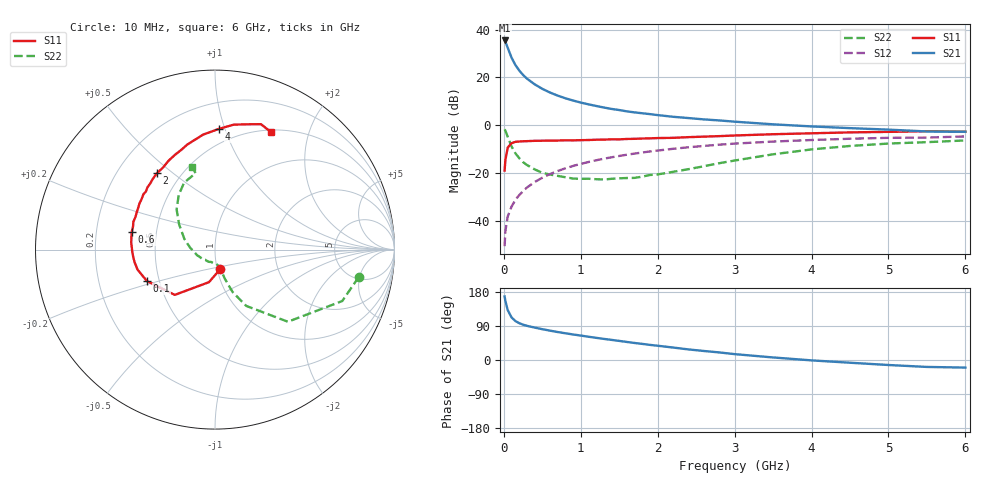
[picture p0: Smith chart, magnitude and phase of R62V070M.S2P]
! SIEMENS Small Signal Semiconductors
! BFR193
! Si NPN RF Bipolar Junction Transistor in SOT23
! VCE = 2 V  IC = 70 mA
! Common Emitter S-Parameters:  May  1996
# GHz  S  MA  R  50
!  f  S11  S21  S12  S22
! GHz  MAG  ANG  MAG  ANG  MAG  ANG  MAG  ANG
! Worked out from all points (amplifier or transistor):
!   36 points, 10 MHz to 6 GHz, reference 50 ohm
!   highest |S21| = 35.5 dB at 10 MHz (marker M1)
!   |S21| within 3 dB of that: start of sweep to 49.59 MHz
!   unconditionally stable (mu >= 1): 227.5 MHz to 2.247 GHz
!   at 250 MHz: K = 1.01, MAG = 23.6 dB, |S12| = -27.7 dB
!   at 1.4 GHz: K = 1.03, MAG = 9.0 dB, |S12| = -13.5 dB
!   at 6 GHz: K = 0.98, MSG = 1.0 dB, |S12| = -4.7 dB
!   S11 on the Smith chart (normalised r, x): 10 MHz: 1.04, -0.23; 100 MHz: 0.43, -0.18; 600 MHz: 0.36, +0.09; 2 GHz: 0.37, +0.44; 4 GHz: 0.39, +0.96; 6 GHz: 0.52, +1.45
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0.01  0.1114 -74.2  59.45 167.6  0.0029 79.5  0.8152 -10.8
0.02  0.1843 -100.4  56.14 156.1  0.006 72.3  0.7648 -22.0
0.05  0.3373 -131.6  41.92 131.8  0.0121 69.0  0.5715 -44.7
0.1  0.4179 -155.2  25.99 112.4  0.0195 69.5  0.3586 -61.0
0.15  0.4456 -165.5  18.21 102.8  0.0271 71.9  0.2568 -67.4
0.2  0.4536 -171.1  13.97 97.2  0.0341 74.3  0.2032 -69.6
0.25  0.4578 -175.2  11.25 93.2  0.0413 74.9  0.1675 -71.5
0.3  0.461 -178.6  9.426 90.2  0.0491 75.7  0.1462 -72.3
0.4  0.4683 175.3  7.171 85.6  0.0641 75.6  0.1181 -74.1
0.5  0.4705 172.1  5.76 81.3  0.0788 75.1  0.1001 -75.4
0.6  0.4743 167.9  4.817 77.5  0.094 73.9  0.0919 -77.7
0.7  0.4744 164.2  4.149 73.8  0.109 72.9  0.0863 -81.1
0.8  0.4804 161.3  3.65 70.5  0.1243 71.5  0.0806 -84.5
1.1  0.4868 151.6  2.724 61.4  0.1685 67.4  0.075 -97.5
1.6  0.512 137.3  1.938 47.6  0.2396 59.5  0.0778 -128.2
2  0.5346 127.2  1.621 37.6  0.2929 53.0  0.0925 -152.5
2.2  0.5409 122.5  1.494 32.9  0.3187 49.7  0.1049 -162.9
3.5  0.6439 95.9  1.039 6.7  0.4516 28.1  0.2443 144.9
4  0.6733 88.1  0.938 -1.0  0.4869 20.9  0.3096 133.7
4.5  0.7039 81.5  0.864 -7.2  0.518 13.8  0.3654 123.6
5.5  0.7441 69.9  0.735 -18.3  0.5476 0.2  0.4393 104.2
6  0.7264 64.8  0.726 -20.0  0.5791 -3.8  0.4771 105.6
